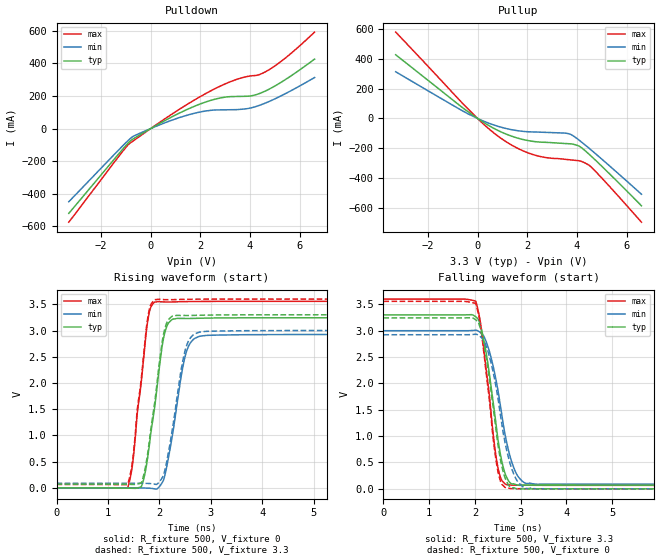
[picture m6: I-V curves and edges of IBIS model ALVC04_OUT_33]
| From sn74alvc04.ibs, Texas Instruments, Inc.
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[Model]   ALVC04_OUT_33
Model_type  Output
Vref =   0
Rref =   500
Cref =   50p
Vmeas =   1.5
| variable   typ   min   max
C_comp   5.94pF   4.11pF   9.05pF
| C_pullup   6.48pF   4.13pF   9.05pF
| C_pulldown   5.39pF   4.11pF   7.73pF
[Temperature Range]   40   100   -40
| Ambient temperature   25   85   -40
[Voltage range]   3.3   3   3.6
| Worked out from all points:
|   slope of the pulldown table from 0 to 0.495 V, typ, clamps not added: 11.6 ohm
|   slope of the pullup table from 0 to 0.495 V, typ, clamps not added: 9.56 ohm
|   rising waveform, R_fixture 500, V_fixture 0: 20-80 % time 256ps typ, 286ps min, 224ps max; typ from 0 V to 3.24 V
|   falling waveform, R_fixture 500, V_fixture 3.3: 20-80 % time 315ps typ, 378ps min, 276ps max; typ from 3.3 V to 0.073 V
|   rising waveform, R_fixture 500, V_fixture 3.3: 20-80 % time 254ps typ, 280ps min, 223ps max; typ from 0.073 V to 3.3 V
|   falling waveform, R_fixture 500, V_fixture 0: 20-80 % time 312ps typ, 369ps min, 274ps max; typ from 3.24 V to 0 V
[Pulldown]
| ALVC04_OUT_33
|   Voltage   I(typ)   I(min)   I(max)
-3.3V     -520mA     -448.7mA   -574.2mA
-1.115V   -124.2mA   -103.8mA   -136.8mA
-905mV    -88.36mA   -72.48mA   -98.82mA
-720mV    -64.47mA   -49.14mA   -77.2mA
840mV     70.73mA    50.73mA    87.26mA
2.07V     155.1mA    103.9mA    202.4mA
2.94V     191.4mA    114.9mA    270mA
3.87V     198.2mA    121.8mA    318.7mA
4.33V     212.1mA    139.8mA    328.8mA
4.755V    240.6mA    165.1mA    359.8mA
5.54V     311.9mA    223.3mA    446.9mA
6.6V      426mA      313mA      591.6mA
[Pullup]
| ALVC04_OUT_33
|   Voltage   I(typ)   I(min)   I(max)
-3.3V     425.7mA    312.1mA    577.2mA
-485mV    56.93mA    39.54mA    80.6mA
200mV     -22.13mA   -14.87mA   -31.9mA
715mV     -71.46mA   -46.96mA   -104.7mA
1.465V    -123.7mA   -77.88mA   -186.7mA
2.215V    -152.8mA   -90.11mA   -240.3mA
2.78V     -159.7mA   -93.2mA    -262.1mA
3.615V    -168.3mA   -100.1mA   -274.6mA
4.09V     -185.4mA   -145.2mA   -282.8mA
4.44V     -231.4mA   -192.2mA   -307.5mA
4.63V     -260.4mA   -218.7mA   -333.6mA
6.6V      -583.6mA   -506.4mA   -693.2mA
[Ramp]
| ALVC04_OUT_33
| variable   typ   min   max
dV/dt_r   1.95/2.60E-10   1.77/2.93E-10   2.14/2.30E-10
dV/dt_f   1.94/3.17E-10   1.75/3.89E-10   2.12/2.78E-10
R_load = 500
[Rising Waveform]
| ALVC04_OUT_33
R_fixture =   500
C_fixture =   0
L_fixture =   0
V_fixture =   0
V_fixture_min = 0
V_fixture_max = 0
|   Time   V(typ)   V(min)   V(max)
0s        40.08pV    3.859nV    33pV
1.38ns    -3.883mV   350uV      -1.692mV
1.48ns    -5.935mV   443.1uV    457.9mV
1.685ns   128.3mV    -1.223mV   2.373V
1.81ns    845.3mV    -4.447mV   3.368V
1.975ns   2.088V     -1.409mV   3.552V
2.16ns    3.113V     486.3mV    3.544V
2.525ns   3.23V      2.588V     3.552V
2.915ns   3.237V     2.908V     3.555V
40ns      3.243V     2.924V     3.557V
[Falling Waveform]
| ALVC04_OUT_33
R_fixture =   500
C_fixture =   0
L_fixture =   0
V_fixture =   3.3
V_fixture_min = 3
V_fixture_max = 3.6
|   Time   V(typ)   V(min)   V(max)
0s        3.3V       3V         3.6V
2.02ns    3.263V     3.01V      3.557V
2.115ns   3.12V      2.969V     3.189V
2.205ns   2.777V     2.876V     2.574V
2.485ns   1.068V     1.96V      494.6mV
2.575ns   580mV      1.483V     183.5mV
2.705ns   200.6mV    841.3mV    77.51mV
2.955ns   68.1mV     222mV      69.15mV
3.365ns   73.05mV    87.66mV    67.86mV
40ns      72.86mV    89.69mV    66.1mV
[Rising Waveform]
| ALVC04_OUT_33
R_fixture =   500
C_fixture =   0
L_fixture =   0
V_fixture =   3.3
V_fixture_min = 3
V_fixture_max = 3.6
|   Time   V(typ)   V(min)   V(max)
0s        72.86mV    89.69mV    66.1mV
1.38ns    69.16mV    89.97mV    64.65mV
1.48ns    67.22mV    90.03mV    524.9mV
1.685ns   202.6mV    88.31mV    2.436V
1.81ns    925.7mV    85.07mV    3.419V
1.975ns   2.176V     88.94mV    3.596V
2.155ns   3.171V     558.6mV    3.588V
2.52ns    3.287V     2.682V     3.595V
2.905ns   3.294V     2.984V     3.599V
40ns      3.3V       3V         3.6V
[Falling Waveform]
| ALVC04_OUT_33
R_fixture =   500
C_fixture =   0
L_fixture =   0
V_fixture =   0
V_fixture_min = 0
V_fixture_max = 0
|   Time   V(typ)   V(min)   V(max)
0s        3.243V     2.924V     3.557V
2.02ns    3.205V     2.934V     3.513V
2.115ns   3.058V     2.89V      3.14V
2.2ns     2.73V      2.803V     2.553V
2.48ns    1V         1.845V     444.5mV
2.575ns   486.9mV    1.307V     113.7mV
2.705ns   119.8mV    696mV      11.03mV
2.95ns    -4.394mV   121mV      2.699mV
3.36ns    34.51uV    115.1uV    1.693mV
40ns      40.02pV    3.859nV    33.05pV
